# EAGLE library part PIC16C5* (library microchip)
MICROCONTROLLER EPROM/ROM-based
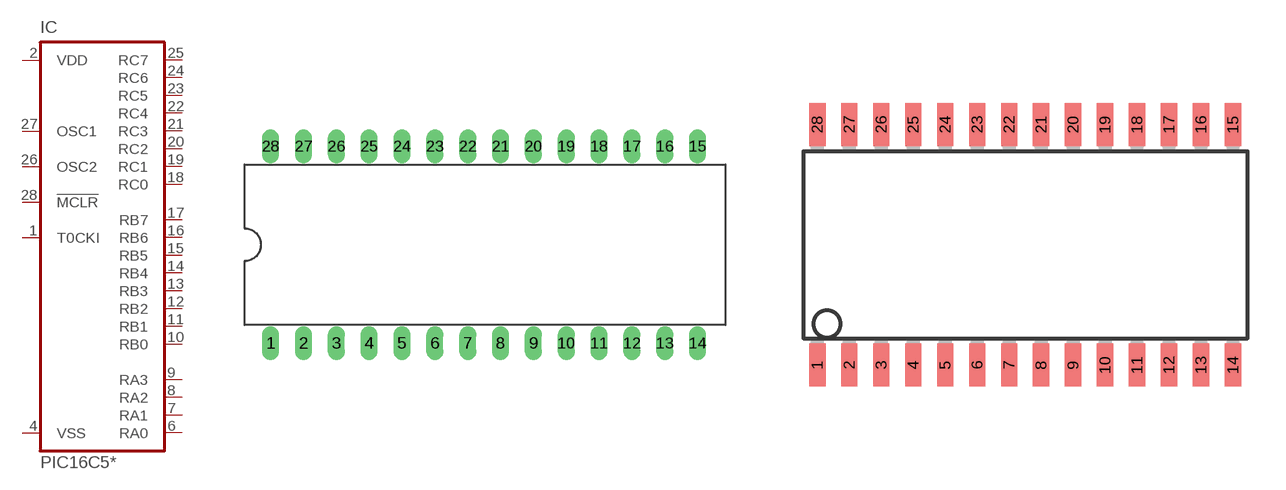
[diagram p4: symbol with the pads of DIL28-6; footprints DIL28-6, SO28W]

Designator prefix IC

## PIC16C55P (MF: MICROCHIP; MPN: PIC16C55-LPI/P; OC_FARNELL: 9759271; OC_NEWARK: 23C3344), PIC16C57P (MF: MICROCHIP; MPN: PIC16C57-HS/P; OC_FARNELL: 1523927; OC_NEWARK: 61K3440), PIC16C57AP (MF: MICROCHIP; MPN: PIC16C57-HS/P; OC_FARNELL: 1084260; OC_NEWARK: 61K3440)  [DIL28-6]
1  T0CKI  in
2  VDD  pwr
3  NC  nc
4  VSS  pwr
5  NC  nc
6  RA0
7  RA1
8  RA2
9  RA3
10  RB0
11  RB1
12  RB2
13  RB3
14  RB4
15  RB5
16  RB6
17  RB7
18  RC0
19  RC1
20  RC2
21  RC3
22  RC4
23  RC5
24  RC6
25  RC7
26  OSC2  out
27  OSC1  in
28  !MCLR  in

## PIC16C55SO (MF: MICROCHIP; MPN: PIC16C55A-04/SO; OC_FARNELL: 9759280; OC_NEWARK: 96K3793), PIC16C57SO (MF: MICROCHIP; MPN: PIC16C57-HS/SO; OC_FARNELL: 9759395; OC_NEWARK: 23C3614), PIC16C57ASO (MF: MICROCHIP; MPN: PIC16C57-XTI/P; OC_FARNELL: 9759395; OC_NEWARK: 88K1971)  [SO28W]
Pads as for DIL28-6

## PIC16C55SS (MF: MICROCHIP; MPN: PIC16C55A-20E/SS; OC_FARNELL: unknown; OC_NEWARK: 23C3402), PIC16C57SS (MF: MICROCHIP; MPN: PIC16C57C-04I/SS; OC_FARNELL: unknown; OC_NEWARK: 23C3683), PIC16C57ASS (MF: MICROCHIP; MPN: PIC16C57C-04I/SS; OC_FARNELL: unknown; OC_NEWARK: 23C3683)  [SSOP28]
Pads as for DIL28-6

## Footprint DIL28-6 (pad centres in mm)
Dual In Line package type P
drill 0.813 long: 1 -16.51,-7.62; 2 -13.97,-7.62; 3 -11.43,-7.62; 4 -8.89,-7.62; 5 -6.35,-7.62; 6 -3.81,-7.62; 7 -1.27,-7.62; 8 1.27,-7.62; 9 3.81,-7.62; 10 6.35,-7.62; 11 8.89,-7.62; 12 11.43,-7.62; 13 13.97,-7.62; 14 16.51,-7.62; 15 16.51,7.62; 16 13.97,7.62; 17 11.43,7.62; 18 8.89,7.62; 19 6.35,7.62; 20 3.81,7.62; 21 1.27,7.62; 22 -1.27,7.62; 23 -3.81,7.62; 24 -6.35,7.62; 25 -8.89,7.62; 26 -11.43,7.62; 27 -13.97,7.62; 28 -16.51,7.62

## Footprint SO28W (pad centres in mm)
28-Lead Plastic Small Outline (SO) Wide, 300 mil Body (SOIC) Source: http://ww1.microchip.com/downloads/en/devicedoc/39632c.pdf
smd 0.65 x 1.7: 1 -7.62,-4.78; 2 -6.35,-4.78; 3 -5.08,-4.78; 4 -3.81,-4.78; 5 -2.54,-4.78; 6 -1.27,-4.78; 7 0,-4.78; 8 1.27,-4.78; 9 2.54,-4.78; 10 3.81,-4.78; 11 5.08,-4.78; 12 6.35,-4.78; 13 7.62,-4.78; 14 8.89,-4.78; 15 8.89,4.78; 16 7.62,4.78; 17 6.35,4.78; 18 5.08,4.78; 19 3.81,4.78; 20 2.54,4.78; 21 1.27,4.78; 22 0,4.78; 23 -1.27,4.78; 24 -2.54,4.78; 25 -3.81,4.78; 26 -5.08,4.78; 27 -6.35,4.78; 28 -7.62,4.78

## Footprint SSOP28 (pad centres in mm)
Shrink Small Outline Package package type SS
smd 0.4 x 1.5: 1 -4.225,-3.625; 2 -3.575,-3.625; 3 -2.925,-3.625; 4 -2.275,-3.625; 5 -1.625,-3.625; 6 -0.975,-3.625; 7 -0.325,-3.625; 8 0.325,-3.625; 9 0.975,-3.625; 10 1.625,-3.625; 11 2.275,-3.625; 12 2.925,-3.625; 13 3.575,-3.625; 14 4.225,-3.625; 15 4.225,3.625; 16 3.575,3.625; 17 2.925,3.625; 18 2.275,3.625; 19 1.625,3.625; 20 0.975,3.625; 21 0.325,3.625; 22 -0.325,3.625; 23 -0.975,3.625; 24 -1.625,3.625; 25 -2.275,3.625; 26 -2.925,3.625; 27 -3.575,3.625; 28 -4.225,3.625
